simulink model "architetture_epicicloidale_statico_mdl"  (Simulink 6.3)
settings: Solver=ode45  StartTime=0.0  StopTime=3  RelTol=1e-3
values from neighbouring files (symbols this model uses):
  bm = 0.8*N*metri*secondo/rad    (= 0.8)    [architetture_epicicloidale_statico.m]    (also in architetture_HEV_startstop_1.m; architetture_HEV_startstop_2.m = 0.08; architetture_epicicloidale.m; architetture_epicicloidale_cont.m)
  I_m = eye(m-1)    [architetture_epicicloidale_statico.m]    (also in architetture_HEV_startstop_1.m; architetture_HEV_startstop_2.m; architetture_epicicloidale.m; architetture_epicicloidale_cont.m)
  Iw0 = 0*wI0    [architetture_epicicloidale_statico.m]    (also in architetture_HEV_startstop_1.m; architetture_HEV_startstop_2.m; architetture_epicicloidale.m; architetture_epicicloidale_cont.m = wI0)
  Jm = 1.6*kg*metri^2    (= 1.6)    [architetture_epicicloidale_statico.m]    (also in architetture_HEV_startstop_1.m = 0.529459095518; architetture_HEV_startstop_2.m = 0.529459095518; architetture_epicicloidale.m; architetture_epicicloidale_cont.m)
  Jr = Jr([1:m-1],[1:m-1])    [architetture_epicicloidale_statico.m]    (also in architetture_HEV_startstop_1.m; architetture_HEV_startstop_2.m; architetture_epicicloidale.m; architetture_epicicloidale_cont.m)
  Kf = diag(diag(MLb)'./fliplr(tau_m(1:m-1)))    [architetture_epicicloidale_statico.m]    (also in architetture_HEV_startstop_1.m; architetture_HEV_startstop_2.m; architetture_epicicloidale_cont.m; architetture_epicicloidale_HEV.m)
  Kr = Kr([1:m-1])    [architetture_epicicloidale_statico.m]    (also in architetture_HEV_startstop_1.m; architetture_HEV_startstop_2.m; architetture_epicicloidale.m; architetture_epicicloidale_cont.m)
  Li = 0.1*Henry    (= 0.1)    [architetture_epicicloidale_statico.m]    (also in architetture_HEV_startstop_1.m; architetture_HEV_startstop_2.m; architetture_epicicloidale.m; architetture_epicicloidale_cont.m)
  m = 5    [architetture_epicicloidale_statico.m]    (also in architetture_HEV_startstop_1.m; architetture_HEV_startstop_2.m; CVT_New.m = 1; CVT_New_th.m = 1)
  Mi = 0.08*Henry    (= 0.08)    [architetture_epicicloidale_statico.m]    (also in architetture_HEV_startstop_1.m; architetture_HEV_startstop_2.m; architetture_epicicloidale.m; architetture_epicicloidale_cont.m)
  MKr = MKr([1:m-1],[1:m-1])    [architetture_epicicloidale_statico.m]    (also in architetture_HEV_startstop_1.m; architetture_HEV_startstop_2.m; architetture_epicicloidale.m; architetture_epicicloidale_cont.m)
  MLb = MLb([1:m-1],[1:m-1])    [architetture_epicicloidale_statico.m]    (also in architetture_HEV_startstop_1.m; architetture_HEV_startstop_2.m; architetture_epicicloidale.m; architetture_epicicloidale_cont.m)
  MR = MR([1:m-1],[1:m-1])    [architetture_epicicloidale_statico.m]    (also in architetture_HEV_startstop_1.m; architetture_HEV_startstop_2.m; architetture_epicicloidale.m; architetture_epicicloidale_cont.m)
  Nar = 200    [architetture_epicicloidale_statico.m]    (also in architetture_HEV_startstop_1.m; architetture_HEV_startstop_2.m; architetture_epicicloidale.m; architetture_epicicloidale_cont.m)
  Nc = 30    [architetture_epicicloidale_statico.m]    (also in architetture_HEV_startstop_1.m; architetture_HEV_startstop_2.m; architetture_epicicloidale.m; architetture_epicicloidale_cont.m)
  p = 1    [architetture_epicicloidale_statico.m]    (also in architetture_HEV_startstop_1.m; architetture_HEV_startstop_2.m; architetture_epicicloidale.m; architetture_epicicloidale_cont.m)
  Phir = 0.02*Weber    (= 0.02)    [architetture_epicicloidale_statico.m]    (also in architetture_HEV_startstop_1.m; architetture_HEV_startstop_2.m; architetture_epicicloidale.m; architetture_epicicloidale_cont.m)
  r_r = xds*Nr/(2*pi)    (= 0.248281711223)    [architetture_epicicloidale_statico.m]    (also in architetture_HEV_startstop_1.m; architetture_HEV_startstop_2.m; architetture_epicicloidale_HEV.m; architetture_HEV_controllo.m)
  r_s = r_r-2*r_p    (= 0.101859163579)    [architetture_epicicloidale_statico.m]    (also in architetture_HEV_startstop_1.m; architetture_HEV_startstop_2.m; architetture_epicicloidale.m = 0.0732112738223; architetture_epicicloidale_cont.m = 0.0732112738223)
  Ri = 3*Ohm    (= 3)    [architetture_epicicloidale_statico.m]    (also in architetture_HEV_startstop_1.m = 0.1; architetture_HEV_startstop_2.m = 0.1; architetture_epicicloidale.m; architetture_epicicloidale_cont.m)
  Star = Si    [architetture_epicicloidale_statico.m]    (also in architetture_HEV_startstop_1.m; architetture_HEV_startstop_2.m; architetture_epicicloidale.m; architetture_epicicloidale_cont.m)
  Tc = 0.05*ms    (= 5e-05)    [architetture_epicicloidale_statico.m]    (also in architetture_HEV_startstop_1.m; architetture_HEV_startstop_2.m; CVT_New.m; CVT_New_th.m)
  Thm0 = 0    [architetture_epicicloidale_statico.m]    (also in architetture_HEV_startstop_1.m; architetture_HEV_startstop_2.m; architetture_epicicloidale.m; architetture_epicicloidale_cont.m)
  tTb = tTb(:,[1:m-1])    [architetture_epicicloidale_statico.m]    (also in architetture_HEV_startstop_1.m; architetture_HEV_startstop_2.m; architetture_epicicloidale.m; architetture_epicicloidale_cont.m)
  W_ice = 20*rad/secondo    (= 20)    [architetture_epicicloidale_statico.m]
  Wc_0 = -0*0.2*rad/secondo    (= 0)    [architetture_epicicloidale_statico.m]    (also in architetture_epicicloidale.m; architetture_epicicloidale_cont.m; architetture_epicicloidale_HEV.m; architetture_epicicloidale_prova.m)
  Wm0 = 0*Wr_d    (= 0)    [architetture_epicicloidale_statico.m]    (also in architetture_HEV_startstop_1.m; architetture_HEV_startstop_2.m; architetture_epicicloidale.m; architetture_epicicloidale_cont.m = 62.5)
  Wr_0 = WW_0(5),    [CVT_New.m]    (also in CVT_New_th.m; architetture_epicicloidale.m = Sys1.C(3,:)*[Wc_0; Wsc_0]; Confronto_CVT_EMR.m = 0; epicicloidale.m = Sys1.C(3,:)*[Wc_0; Wsc_0])
  Ws_0 = 0*0.1*rad/secondo    (= 0)    [architetture_epicicloidale_statico.m]    (also in epicicloidale_confronto_statico_elastico.m = 0.1; epicicloidale_statico.m = 0.1)
undefined symbols (not defined in the file or in its folder): a_0, a_1, B_Pneumatico, DFKc_max, eps_sk, K_Pneumatico, Lambda_mu, Mass_Matrix, Massa_Corpo_Auto, Mu_lambda, Raggio_Ruota_Ant, Raggio_Ruota_Pos, T_omega, tau_a0
libraries: simulink x11, dspmtrx3 x4, Tire_Soil x2, POG_Sincronous_Motors x1

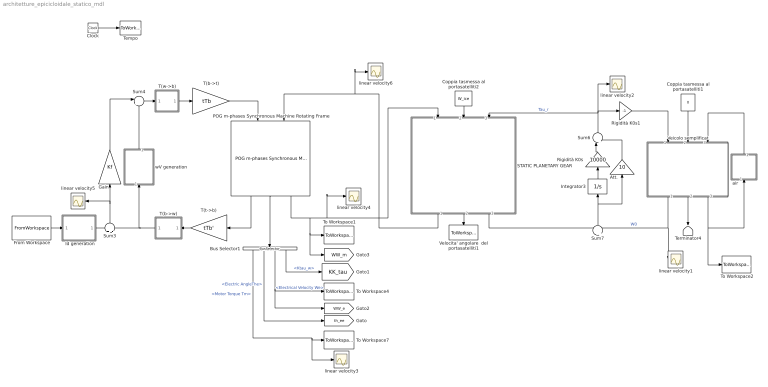
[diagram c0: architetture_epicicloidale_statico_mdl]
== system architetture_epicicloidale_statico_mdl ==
  " Id generation" : Subsystem
  Att. : Gain  Orientation=up  Gain=10
  Bus Selector1 : BusSelector  Orientation=down  OutputSignals=Motor Torque Tm,Electric AngleThe,Electrical Velocity We,Ktau_w
  Clock : Clock
  Coppia tasmessa al portasatelliti1 : Constant  Orientation=down  Value=0
  Coppia tasmessa al portasatelliti2 : Constant  Orientation=down  Value=W_ice
  From Workspace : FromWorkspace  VariableName=[T_in Tau_des]  SampleTime=0
  Gain : Gain  Orientation=up  Gain=Kf  Multiplication=Matrix(K*u) (u vector)
  Integrator3 : Integrator  Orientation=up
  POG m-phases Synchronous Machine Rotating Frame : POG_Sincronous_Motors/POG m-phases Synchronous Machine Rotating Frame  Orientation=down  Motor_Par=[m p]  Phase_Par=[Nc Star]  Electric_Par=[Ri Li Mi]  Mech_Par=[Jm bm]  Plux_Par=[Phir Nar]  Iniz_Cond=[Wm0; Thm0; Iw0]  TipoFlux=User defined  Tipo=Tipo  alfa=al  degree=6  TipoF=Tipo
  Rigidità K0s : Gain  Orientation=up  Gain=10000
  Rigidità K0s1 : Gain  Gain=-1
  STATIC PLANETARY GEAR : Subsystem  Orientation=down  mask(POG Gruppo epicicloidale){Raggi_sun_ring=[r_s, r_r], Tipo_di_Modello=Modello ridotto Ws-Wc, Cond_in_Ws_Wc=[Ws_0,  Wc_0], Cond_in_Wc_Wr=[Wc_0,  Wr_0], Cond_in_Ws_Wr=[Ws_0,  Wr_0], Cond_in=[Ws_0, Wc_0, Wr_0]}
      mask prompts: Raggi_sun_ring "Raggi Sun, Ring: [r_s, r_r]-->[m,m]"; Tipo_di_Modello "Tipo di modello"; Cond_in_Ws_Wc "Condizioni iniziali: [Ws_0,  Wc_0]-->[rad/s]"; Cond_in_Wc_Wr "Condizioni iniziali: [Wc_0,  Wr_0]-->[rad/s]"; Cond_in_Ws_Wr "Condizioni iniziali: [Ws_0,  Wr_0]-->[rad/s]"; Cond_in "Condizioni iniziali: [Ws_0,  Wc_0, Wr_0]-->[rad/s]"
      mask help: Gruppo epicicloidale: [r_s, r_r]= Raggi di: sun e ring; [Ws_0, Wc_0, Wr_0]=Velocita' iniziali di sun, carrieri, ring;
      mask init:
      | r_s=Raggi_sun_ring(1);
      | r_r=Raggi_sun_ring(2);
      | 
      | %
      | %%%%%%%%%%%%%%%%%%%%%%%%%%%%%%%%%%%%%%%%%%%%%%%%%%%%%%%%%%%%%%%%%%%%%%%%%%%
      | %   Modello statico tutti i casi
      | %%%%%%%%%%%%%%%%%%%%%%%%%%%%%%%%%%%%%%%%%%%%%%%%%%%%%%%%%%%%%%%%%%%%%%%%%%%
      | if Tipo_di_Modello=='Modello ridotto Ws-Wc'
      |       %
      |     B= [ -1/r_r*r_s,  (r_s+r_r)/r_r];
      |     %
      |     Ws_0=double(Cond_in_Ws_Wc(1));
      |     Wc_0=double(Cond_in_Ws_Wc(2));
      |     We_0=[Ws_0 Wc_0];
      |     %
      | elseif Tipo_di_Modello=='Modello ridotto Wc-Wr'
      |     B= [ (r_s+r_r)/r_s,  -1/r_s*r_r];
      |    %
      |     Wc_0=double(Cond_in_Wc_Wr(1));
      |     Wr_0=double(Cond_in_Wc_Wr(2));
      |     We_0=[Wc_0 Wr_0];
      |     %
      | elseif Tipo_di_Modello=='Modello ridotto Ws-Wr'
      |  
      |     B=[1/(r_s+r_r)*r_s, 1/(r_s+r_r)*r_r];
      |    %
      |     Ws_0=double(Cond_in_Ws_Wr(1));
      |     Wr_0=double(Cond_in_Ws_Wr(2));
      |     We_0=[Ws_0 Wr_0];
      | end
  Sum3 : Sum  Orientation=up  Inputs=+|-
  Sum4 : Sum  Inputs=|++
  Sum6 : Sum  Orientation=up  Inputs=|++
  Sum7 : Sum  Orientation=up  Inputs=-|+
  T(b->t) : Gain  Gain=tTb  Multiplication=Matrix(K*u) (u vector)
  T(b->w) : Subsystem  Orientation=left  AncestorBlock=|
      | POG_Electric_Bloks/POG m-phases
      | Synchronous Machine
      | Rotating Frame/T(b->w)
  T(t->b) : Gain  Orientation=left  Gain=tTb'  Multiplication=Matrix(K*u) (u vector)
  T(w->b) : Subsystem  AncestorBlock=|
      | POG_Electric_Bloks/POG m-phases
      | Synchronous Machine
      | Rotating Frame/T(w->b)
  Tempo : ToWorkspace  VariableName=t  SampleTime=Tc  SaveFormat=Array
  Terminator4 : Terminator
  To Workspace1 : ToWorkspace  VariableName=Wm  SampleTime=Tc  SaveFormat=Array
  To Workspace2 : ToWorkspace  VariableName=Vvehicle  SampleTime=Tc  SaveFormat=Array
  To Workspace4 : ToWorkspace  VariableName=We  SampleTime=Tc  SaveFormat=Array
  To Workspace7 : ToWorkspace  VariableName=Tm  SampleTime=Tc  SaveFormat=Array
  Veicolo semplificat : Subsystem  Orientation=down
  Velocita' angolare  del portasatelliti1 : ToWorkspace  VariableName=Tau_ice  SampleTime=Tc  SaveFormat=Array
  air : Subsystem  Orientation=up
  linear velocity{1..6} (6 alike) : Scope
  wV generation : Subsystem  Orientation=up
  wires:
  Clock/1 -> Tempo/1
  POG m-phases Synchronous Machine Rotating Frame/3 -> To Workspace1/1, [WW_m], STATIC PLANETARY GEAR/1(W1), linear velocity4/1
  POG m-phases Synchronous Machine Rotating Frame/2 -> Bus Selector1/1
  Bus Selector1/3 -> To Workspace4/1, [WW_e]  "<Electrical Velocity We>"
  T(w->b)/1(It) -> T(b->t)/1
  T(b->t)/1 -> POG m-phases Synchronous Machine Rotating Frame/1
  T(t->b)/1 -> T(b->w)/1(Vt)
  T(b->w)/1(Vw) -> wV generation/1(In1), Sum3/2
  POG m-phases Synchronous Machine Rotating Frame/1 -> T(t->b)/1
  Bus Selector1/2 -> [th_ee]  "<Electric AngleThe>"
  Bus Selector1/1 -> To Workspace7/1, linear velocity3/1  "<Motor Torque Tm>"
  Att./1 -> Sum6/2
  Rigidità K0s/1 -> Sum6/1
  Integrator3/1 -> Rigidità K0s/1
  Sum6/1 -> linear velocity2/1, Rigidità K0s1/1, STATIC PLANETARY GEAR/3(Tau3)  "Tau_r"
  Sum7/1 -> Att./1, Integrator3/1
  Coppia tasmessa al portasatelliti1/1 -> Veicolo semplificat/2(Tau2)
  Rigidità K0s1/1 -> Veicolo semplificat/1(Tau1)
  " Id generation"/1(Out1) -> Sum3/1
  Sum3/1 -> Gain/1, linear velocity5/1
  Sum4/1 -> T(w->b)/1(Iw)
  From Workspace/1 -> " Id generation"/1(In1)
  Gain/1 -> Sum4/1
  wV generation/1(Out1) -> Sum4/2
  Veicolo semplificat/1(W1) -> Sum7/2, linear velocity1/1  "W0"
  Veicolo semplificat/3(V) -> To Workspace2/1, air/1(In1)
  Bus Selector1/4 -> [KK_tau]  "<Ktau_w>"
  air/1(Out1) -> Veicolo semplificat/3(Fres)
  Veicolo semplificat/2(W2) -> Terminator4/1
  Coppia tasmessa al portasatelliti2/1 -> STATIC PLANETARY GEAR/2(W2)
  STATIC PLANETARY GEAR/2(Tau2) -> Velocita' angolare  del portasatelliti1/1
  STATIC PLANETARY GEAR/3(W3) -> Sum7/1
  STATIC PLANETARY GEAR/1(Tau1) -> POG m-phases Synchronous Machine Rotating Frame/2, linear velocity6/1

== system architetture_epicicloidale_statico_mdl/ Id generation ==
  In1 : Inport
  Divide : Product  Inputs=*/  OutScaling=2^-10
  Product : Product
  modulo : Subsystem
  versore : Subsystem
  Out1 : Outport
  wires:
  [KK_tau] -> modulo/1(In1), versore/1(In1)
  modulo/1(Out1) -> Divide/2
  Divide/1 -> Product/1
  versore/1(Out1) -> Product/2
  In1/1 -> Divide/1
  Product/1 -> Out1/1

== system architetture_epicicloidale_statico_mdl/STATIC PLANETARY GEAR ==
  W1 : Inport
  W2 : Inport  Port=2
  Tau3 : Inport  Orientation=left  Port=3
  Demux : Demux  Orientation=left  Outputs=2
  Mux : Mux  Inputs=2
  Rsc : Gain  Gain=B  Multiplication=Matrix(K*u)
  Rsc' : Gain  Orientation=left  Gain=B'  Multiplication=Matrix(K*u)
  Tau1 : Outport  Orientation=left
  Tau2 : Outport  Orientation=left  Port=2
  W3 : Outport  Port=3
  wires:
  Demux/2 -> Tau2/1  "Tau2"
  Demux/1 -> Tau1/1  "Tau1"
  Rsc'/1 -> Demux/1
  Mux/1 -> Rsc/1
  W2/1 -> Mux/2  "W2"
  W1/1 -> Mux/1  "W1"
  Rsc/1 -> W3/1  "W3"
  Tau3/1 -> Rsc'/1  "Tau3"

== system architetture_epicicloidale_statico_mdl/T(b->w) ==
  Vt : Inport
  Product : Product  Multiplication=Matrix(*)
  Vw : Outport
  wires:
  Vt/1 -> Product/2
  Product/1 -> Vw/1
  [T_w_be] -> Product/1

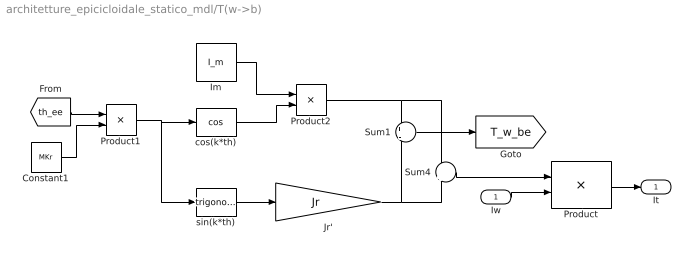
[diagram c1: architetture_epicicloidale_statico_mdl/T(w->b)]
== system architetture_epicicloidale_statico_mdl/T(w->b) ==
  Iw : Inport
  Constant1 : Constant  Value=MKr
  Im : Constant  Value=I_m  VectorParams1D=off
  Jr' : Gain  Gain=Jr  Multiplication=Matrix(K*u)
  Product : Product  Multiplication=Matrix(*)
  Product1 : Product
  Product2 : Product
  Sum1 : Sum  Inputs=+|-
  Sum4 : Sum  Inputs=+|+
  cos(k*th) : Trigonometry  Operator=cos
  sin(k*th) : Trigonometry
  It : Outport
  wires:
  Sum4/1 -> Product/1
  Product/1 -> It/1
  Iw/1 -> Product/2
  Jr'/1 -> Sum4/2, Sum1/2
  Product2/1 -> Sum4/1, Sum1/1
  Im/1 -> Product2/1
  cos(k*th)/1 -> Product2/2
  Product1/1 -> sin(k*th)/1, cos(k*th)/1
  Constant1/1 -> Product1/2
  [th_ee] -> Product1/1
  sin(k*th)/1 -> Jr'/1
  Sum1/1 -> [T_w_be]

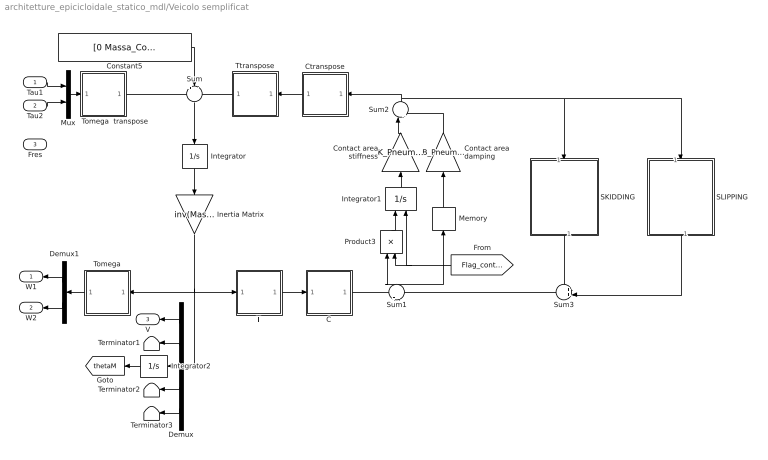
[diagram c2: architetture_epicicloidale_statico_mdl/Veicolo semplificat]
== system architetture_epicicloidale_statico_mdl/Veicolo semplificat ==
  Tau1 : Inport
  Tau2 : Inport  Port=2
  Fres : Inport  Port=3
  C : Subsystem
  Constant5 : Constant  Value=[0 Massa_Corpo_Auto*9.81 0 0 0]
  Contact area damping : Gain  Orientation=up  Gain=B_Pneumatico  Multiplication=Matrix(K*u) (u vector)
  Contact area stiffness : Gain  Orientation=up  Gain=K_Pneumatico  Multiplication=Matrix(K*u) (u vector)
  Ctranspose : Subsystem  Orientation=left
  Demux : Demux  Orientation=left  Outputs=5
  Demux1 : Demux  Orientation=left  Outputs=2
  Inertia Matrix : Gain  Orientation=down  Gain=inv(Mass_Matrix)  Multiplication=Matrix(K*u)
  Integrator : Integrator  Orientation=down  InitialCondition=[0 0 0 0 0]
  Integrator1 : Integrator  Orientation=up  ExternalReset=falling  InitialCondition=[0 0 0 0 0 0]
  Integrator2 : Integrator  Orientation=left
  Memory : Memory  Orientation=up
  Mux : Mux  Inputs=2
  Product3 : Product  Orientation=up  Inputs=**
  SKIDDING : Subsystem  Orientation=down  AncestorBlock=Tire_Soil/Tire-soil contact ENERGETIC/Contatto elastico/SKIDDING
  SLIPPING : Subsystem  Orientation=down  AncestorBlock=Tire_Soil/Tire-soil contact ENERGETIC/Contatto elastico/SLIPPING
  Sum : Sum  Orientation=down  Inputs=+--
  Sum1 : Sum  Orientation=up  Inputs=+-
  Sum2 : Sum  Orientation=up  Inputs=|++
  Sum3 : Sum  Orientation=left  Inputs=++|
  T : Subsystem
  Terminator1 : Terminator
  Terminator2 : Terminator
  Terminator3 : Terminator
  Tomega : Subsystem  Orientation=left
  Tomega  transpose : Subsystem
  Ttranspose : Subsystem  Orientation=left
  W1 : Outport  Orientation=left
  W2 : Outport  Orientation=left  Port=2
  V : Outport  Orientation=left  Port=3
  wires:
  Demux/5 -> Terminator3/1
  Demux/4 -> Terminator2/1
  Demux/2 -> Terminator1/1
  Demux/1 -> V/1
  Tomega/1(Vt) -> Demux1/1
  Tau2/1 -> Mux/2
  Tau1/1 -> Mux/1
  Mux/1 -> Tomega  transpose/1(T)
  Tomega  transpose/1(Tt) -> Sum/1
  Constant5/1 -> Sum/2
  Sum3/1 -> Sum1/2
  SKIDDING/1(Vcsk) -> Sum3/1
  SLIPPING/1(Vcsl) -> Sum3/2
  Memory/1 -> Contact area damping/1
  Integrator1/1 -> Contact area stiffness/1
  Product3/1 -> Integrator1/1
  [Flag_contatto] -> Integrator1/2, Product3/2
  C/1(Xcdot) -> Sum1/1
  Ctranspose/1(F) -> Ttranspose/1(F)
  T/1(Xdot) -> C/1(Xdot)
  Integrator2/1 -> [thetaM]
  Demux/3 -> Integrator2/1
  Contact area stiffness/1 -> Sum2/1
  Contact area damping/1 -> Sum2/2
  Sum1/1 -> Memory/1, Product3/1
  Sum2/1 -> Ctranspose/1(Fc), SLIPPING/1(Fxyz), SKIDDING/1(Fxyz)
  Ttranspose/1(Ft) -> Sum/3
  Inertia Matrix/1 -> T/1(V), Tomega/1(V), Demux/1
  Integrator/1 -> Inertia Matrix/1
  Sum/1 -> Integrator/1
  Demux1/1 -> W1/1
  Demux1/2 -> W2/1

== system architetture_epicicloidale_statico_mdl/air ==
  In1 : Inport  Orientation=up
  air : Fcn  Orientation=up  Expr=10*u^2
  Out1 : Outport  Orientation=up
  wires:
  In1/1 -> air/1
  air/1 -> Out1/1

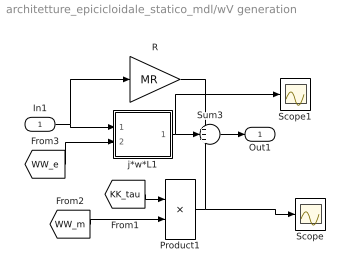
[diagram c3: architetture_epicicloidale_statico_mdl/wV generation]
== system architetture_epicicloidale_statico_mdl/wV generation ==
  In1 : Inport
  Product1 : Product  Multiplication=Matrix(*)
  R : Gain  Gain=MR  Multiplication=Matrix(K*u) (u vector)
  Scope : Scope
  Scope1 : Scope
  Sum3 : Sum  Inputs=+++
  j*w*L1 : Subsystem  AncestorBlock=|
      | POG_Electric_Bloks/POG m-phases
      | Synchronous Machine
      | Rotating Frame/j*w*L
  Out1 : Outport
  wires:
  [KK_tau] -> Product1/1
  [WW_m] -> Product1/2
  R/1 -> Sum3/1
  j*w*L1/1(Out1) -> Sum3/2, Scope1/1
  Product1/1 -> Sum3/3, Scope/1
  In1/1 -> j*w*L1/1(In1), R/1
  Sum3/1 -> Out1/1
  [WW_e] -> j*w*L1/2(In2)

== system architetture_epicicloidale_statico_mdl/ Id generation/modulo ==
  In1 : Inport
  Dot Product : simulink/Math Operations/Dot Product  InputSameDT=on  OutDataType=sfix(16)  OutScaling=2^-10  DoSatur=off
  Math Function : Math  Operator=sqrt
  Out1 : Outport
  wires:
  In1/1 -> Dot Product/1, Dot Product/2
  Dot Product/1 -> Math Function/1
  Math Function/1 -> Out1/1

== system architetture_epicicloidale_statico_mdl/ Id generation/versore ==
  In1 : Inport
  Constant : Constant  Value=0.0001
  Divide : Product  Inputs=*/  OutScaling=2^-10
  Norma  del vettore : Subsystem
  Sum1 : Sum  Inputs=|++
  Out1 : Outport
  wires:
  Divide/1 -> Out1/1  "versore"
  Constant/1 -> Sum1/2
  Sum1/1 -> Divide/2
  Norma  del vettore/1(Out1) -> Sum1/1
  In1/1 -> Norma  del vettore/1(In1), Divide/1

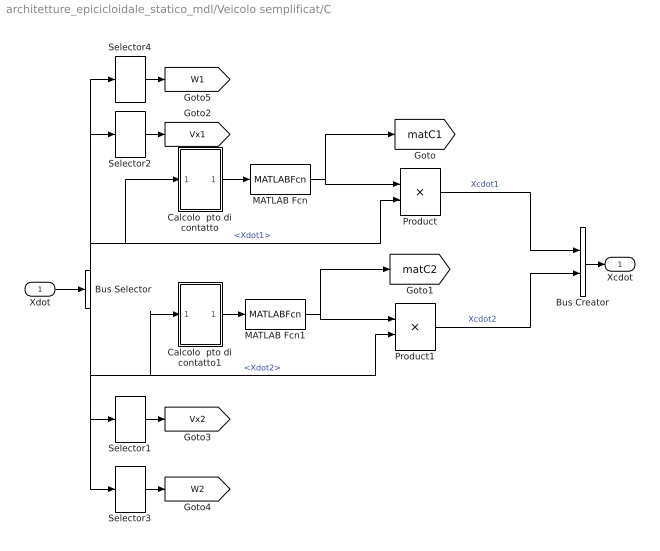
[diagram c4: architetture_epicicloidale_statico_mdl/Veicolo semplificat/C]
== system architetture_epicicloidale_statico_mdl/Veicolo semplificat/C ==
  Xdot : Inport
  Bus Creator : BusCreator  Inputs=2
  Bus Selector : BusSelector  OutputSignals=Xdot1,Xdot2
  Calcolo  pto di contatto : Subsystem
  Calcolo  pto di contatto1 : Subsystem
  MATLAB Fcn : MATLABFcn  MATLABFcn=matrice_c  Output1D=off
  MATLAB Fcn1 : MATLABFcn  MATLABFcn=matrice_c  Output1D=off
  Product : Product  Inputs=**  Multiplication=Matrix(*)
  Product1 : Product  Inputs=**  Multiplication=Matrix(*)
  Selector1 : Selector  InputPortWidth=3
  Selector2 : Selector  InputPortWidth=3
  Selector3 : Selector  Elements=3  InputPortWidth=3
  Selector4 : Selector  Elements=3  InputPortWidth=3
  Xcdot : Outport
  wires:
  Selector3/1 -> [W2]
  Selector4/1 -> [W1]
  Selector1/1 -> [Vx2]
  Selector2/1 -> [Vx1]
  Bus Creator/1 -> Xcdot/1
  Bus Selector/1 -> Selector4/1, Selector2/1, Product/2, Calcolo  pto di contatto/1(In1)  "<Xdot1>"
  Xdot/1 -> Bus Selector/1
  Calcolo  pto di contatto1/1(Out1) -> MATLAB Fcn1/1
  MATLAB Fcn1/1 -> [matC2], Product1/1
  Bus Selector/2 -> Selector3/1, Selector1/1, Calcolo  pto di contatto1/1(In1), Product1/2  "<Xdot2>"
  Product1/1 -> Bus Creator/2  "Xcdot2"
  Calcolo  pto di contatto/1(Out1) -> MATLAB Fcn/1
  MATLAB Fcn/1 -> [matC1], Product/1
  Product/1 -> Bus Creator/1  "Xcdot1"

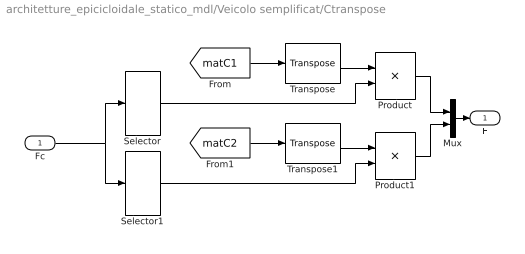
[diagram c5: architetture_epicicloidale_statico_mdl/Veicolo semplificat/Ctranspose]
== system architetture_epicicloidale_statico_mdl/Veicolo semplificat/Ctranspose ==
  Fc : Inport
  Mux : Mux  Inputs=2
  Product : Product  Inputs=**  Multiplication=Matrix(*)
  Product1 : Product  Inputs=**  Multiplication=Matrix(*)
  Selector : Selector  Elements=[1 2 3]  InputPortWidth=6
  Selector1 : Selector  Elements=[4 5 6]  InputPortWidth=6
  Transpose : dspmtrx3/Transpose  Hermitian=off  overflowFlag=on
  Transpose1 : dspmtrx3/Transpose  Hermitian=off  overflowFlag=on
  F : Outport
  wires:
  Selector1/1 -> Product1/2
  Selector/1 -> Product/2
  Fc/1 -> Selector1/1, Selector/1
  Mux/1 -> F/1
  Product1/1 -> Mux/2
  Product/1 -> Mux/1
  [matC2] -> Transpose1/1
  Transpose1/1 -> Product1/1
  [matC1] -> Transpose/1
  Transpose/1 -> Product/1

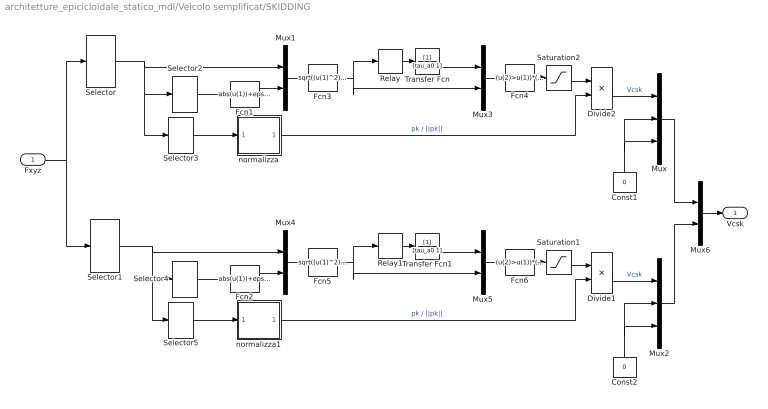
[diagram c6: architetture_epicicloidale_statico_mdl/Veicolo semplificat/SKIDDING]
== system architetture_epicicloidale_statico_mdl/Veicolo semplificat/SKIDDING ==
  Fxyz : Inport
  Const1 : Constant  Orientation=up  Value=0
  Const2 : Constant  Orientation=up  Value=0
  Divide1 : Product  Inputs=**  OutScaling=2^-10
  Divide2 : Product  Inputs=**  OutScaling=2^-10
  Fcn1 : Fcn  Expr=abs(u(1))+eps_sk
  Fcn2 : Fcn  Expr=abs(u(1))+eps_sk
  Fcn3 : Fcn  Expr=sqrt((u(1)^2))/u(4)
  Fcn4 : Fcn  Expr=(u(2)>u(1))*(u(2)-u(1))^2*Kc
  Fcn5 : Fcn  Expr=sqrt((u(1)^2))/u(4)
  Fcn6 : Fcn  Expr=(u(2)>u(1))*(u(2)-u(1))^2*Kc
  Mux : Mux  Inputs=3
  Mux{1,3..6} (5 alike) : Mux  Inputs=2
  Mux2 : Mux  Inputs=3
  Relay : Relay  OnSwitchValue=a_0  OffSwitchValue=a_1  OnOutputValue=a_1  OffOutputValue=a_0
  Relay1 : Relay  OnSwitchValue=a_0  OffSwitchValue=a_1  OnOutputValue=a_1  OffOutputValue=a_0
  Saturation1 : Saturate  UpperLimit=DFKc_max  LowerLimit=0
  Saturation2 : Saturate  UpperLimit=DFKc_max  LowerLimit=0
  Selector : Selector  Elements=[1 2 3]  InputPortWidth=6
  Selector1 : Selector  Elements=[4 5 6]  InputPortWidth=6
  Selector2 : Selector  Elements=[2]  InputPortWidth=3
  Selector3 : Selector  InputPortWidth=3
  Selector4 : Selector  Elements=[2]  InputPortWidth=3
  Selector5 : Selector  InputPortWidth=3
  Transfer Fcn : TransferFcn  Denominator=[tau_a0 1]
  Transfer Fcn1 : TransferFcn  Denominator=[tau_a0 1]
  normalizza : Subsystem
  normalizza1 : Subsystem
  Vcsk : Outport
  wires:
  Mux6/1 -> Vcsk/1
  Mux2/1 -> Mux6/2
  Mux/1 -> Mux6/1
  Const2/1 -> Mux2/3, Mux2/2
  Selector1/1 -> Mux4/1, Selector5/1, Selector4/1
  Divide1/1 -> Mux2/1  "Vcsk"
  Selector4/1 -> Fcn2/1
  Selector5/1 -> normalizza1/1(In1)
  normalizza1/1(Out1) -> Divide1/2  "pk / ||pk||"
  Saturation1/1 -> Divide1/1
  Fcn6/1 -> Saturation1/1
  Fcn5/1 -> Relay1/1, Mux5/2
  Mux4/1 -> Fcn5/1
  Fcn2/1 -> Mux4/2
  Mux5/1 -> Fcn6/1
  Relay1/1 -> Transfer Fcn1/1
  Transfer Fcn1/1 -> Mux5/1
  Const1/1 -> Mux/3, Mux/2
  Selector/1 -> Mux1/1, Selector3/1, Selector2/1
  Divide2/1 -> Mux/1  "Vcsk"
  Fxyz/1 -> Selector1/1, Selector/1
  Selector2/1 -> Fcn1/1
  Selector3/1 -> normalizza/1(In1)
  normalizza/1(Out1) -> Divide2/2  "pk / ||pk||"
  Saturation2/1 -> Divide2/1
  Fcn4/1 -> Saturation2/1
  Fcn3/1 -> Relay/1, Mux3/2
  Mux1/1 -> Fcn3/1
  Fcn1/1 -> Mux1/2
  Mux3/1 -> Fcn4/1
  Relay/1 -> Transfer Fcn/1
  Transfer Fcn/1 -> Mux3/1

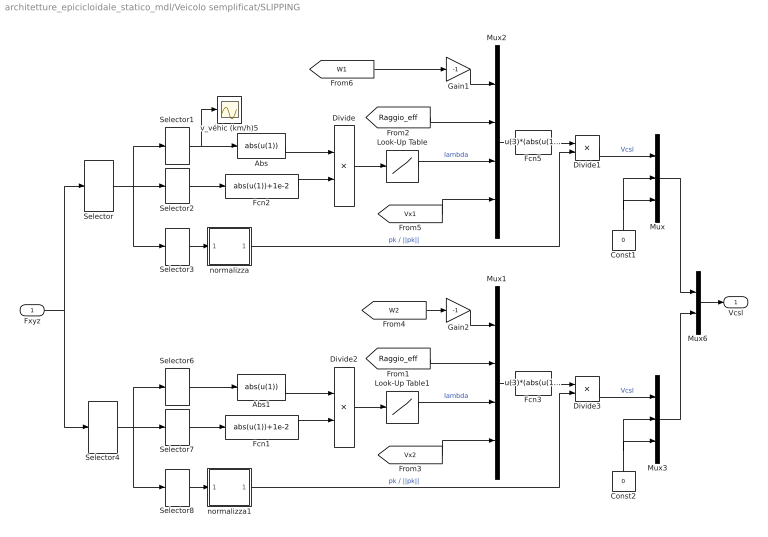
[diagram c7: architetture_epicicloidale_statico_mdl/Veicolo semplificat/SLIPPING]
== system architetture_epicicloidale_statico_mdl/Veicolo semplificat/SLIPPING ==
  Fxyz : Inport
  Abs : Fcn  Expr=abs(u(1))
  Abs1 : Fcn  Expr=abs(u(1))
  Const1 : Constant  Orientation=up  Value=0
  Const2 : Constant  Orientation=up  Value=0
  Divide : Product  Inputs=*/  OutScaling=2^-10
  Divide1 : Product  Inputs=**  OutScaling=2^-10
  Divide2 : Product  Inputs=*/  OutScaling=2^-10
  Divide3 : Product  Inputs=**  OutScaling=2^-10
  Fcn1 : Fcn  Expr=abs(u(1))+1e-2
  Fcn2 : Fcn  Expr=abs(u(1))+1e-2
  Fcn3 : Fcn  Expr=u(3)*(abs(u(1)*u(2))*(abs(u(1)*u(2))<=abs(u(4)))+abs(u(4))*(abs(u(1)*u(2))>abs(u(4))))
  Fcn5 : Fcn  Expr=u(3)*(abs(u(1)*u(2))*(abs(u(1)*u(2))<=abs(u(4)))+abs(u(4))*(abs(u(1)*u(2))>abs(u(4))))
  Gain1 : Gain  Gain=-1
  Gain2 : Gain  Gain=-1
  Look-Up Table : Lookup  InputValues=Mu_lambda  OutputValues=Lambda_mu
  Look-Up Table1 : Lookup  InputValues=Mu_lambda  OutputValues=Lambda_mu
  Mux : Mux  Inputs=3
  Mux1 : Mux
  Mux2 : Mux
  Mux3 : Mux  Inputs=3
  Mux6 : Mux  Inputs=2
  Selector : Selector  Elements=[1 2 3]  InputPortWidth=6
  Selector{1,3,6,8} (4 alike) : Selector  InputPortWidth=3
  Selector2 : Selector  Elements=[2]  InputPortWidth=3
  Selector4 : Selector  Elements=[4 5 6]  InputPortWidth=6
  Selector7 : Selector  Elements=[2]  InputPortWidth=3
  normalizza : Subsystem
  normalizza1 : Subsystem
  v_véhic (km/h)5 : Scope
  Vcsl : Outport
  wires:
  [W2] -> Gain2/1
  [W1] -> Gain1/1
  Mux6/1 -> Vcsl/1
  Mux3/1 -> Mux6/2
  Mux/1 -> Mux6/1
  Const2/1 -> Mux3/3, Mux3/2
  Divide3/1 -> Mux3/1  "Vcsl"
  Const1/1 -> Mux/2, Mux/3
  Divide1/1 -> Mux/1  "Vcsl"
  normalizza1/1(Out1) -> Divide3/2  "pk / ||pk||"
  Selector4/1 -> Selector6/1, Selector8/1, Selector7/1
  Selector7/1 -> Fcn1/1
  Selector8/1 -> normalizza1/1(In1)
  Fcn1/1 -> Divide2/2
  Abs1/1 -> Divide2/1
  Selector6/1 -> Abs1/1
  Look-Up Table1/1 -> Mux1/3  "lambda"
  Divide2/1 -> Look-Up Table1/1
  [Raggio_eff] -> Mux1/2
  Gain2/1 -> Mux1/1
  [Vx2] -> Mux1/4
  Mux1/1 -> Fcn3/1
  Fcn3/1 -> Divide3/1
  Fxyz/1 -> Selector4/1, Selector/1
  normalizza/1(Out1) -> Divide1/2  "pk / ||pk||"
  Selector/1 -> Selector1/1, Selector3/1, Selector2/1
  Selector2/1 -> Fcn2/1
  Selector3/1 -> normalizza/1(In1)
  Fcn2/1 -> Divide/2
  Abs/1 -> Divide/1
  Selector1/1 -> v_véhic (km/h)5/1, Abs/1
  Look-Up Table/1 -> Mux2/3  "lambda"
  Divide/1 -> Look-Up Table/1
  [Raggio_eff] -> Mux2/2
  Gain1/1 -> Mux2/1
  [Vx1] -> Mux2/4
  Mux2/1 -> Fcn5/1
  Fcn5/1 -> Divide1/1

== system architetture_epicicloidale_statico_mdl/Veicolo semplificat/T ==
  V : Inport
  Bus Creator : BusCreator  Inputs=2
  MATLAB Fcn : MATLABFcn  MATLABFcn=matrice_T  Output1D=off
  Product : Product  Inputs=**  Multiplication=Matrix(*)
  Selector : Selector  Elements=[1 2 3]  InputPortWidth=6
  Selector1 : Selector  Elements=[4 5 6]  InputPortWidth=6
  Xdot : Outport
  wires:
  Bus Creator/1 -> Xdot/1
  Selector/1 -> Bus Creator/1  "Xdot1"
  Selector1/1 -> Bus Creator/2  "Xdot2"
  Product/1 -> Selector1/1, Selector/1
  MATLAB Fcn/1 -> [matT], Product/1
  V/1 -> Product/2
  [thetaM] -> MATLAB Fcn/1

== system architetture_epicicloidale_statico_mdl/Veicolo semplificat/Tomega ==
  V : Inport
  Constant5 : Constant  Value=T_omega
  Product : Product  Inputs=**  Multiplication=Matrix(*)
  Vt : Outport
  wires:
  Product/1 -> Vt/1
  V/1 -> Product/2
  Constant5/1 -> Product/1

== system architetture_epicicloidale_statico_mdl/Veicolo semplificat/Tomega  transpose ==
  T : Inport
  Constant5 : Constant  Value=T_omega
  Product : Product  Inputs=**  Multiplication=Matrix(*)
  Transpose : dspmtrx3/Transpose  Hermitian=off  overflowFlag=on
  Tt : Outport
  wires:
  Transpose/1 -> Product/1
  Constant5/1 -> Transpose/1
  T/1 -> Product/2
  Product/1 -> Tt/1

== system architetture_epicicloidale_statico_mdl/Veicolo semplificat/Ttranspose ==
  F : Inport
  Product : Product  Inputs=**  Multiplication=Matrix(*)
  Transpose : dspmtrx3/Transpose  Hermitian=off  overflowFlag=on
  Ft : Outport
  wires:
  Transpose/1 -> Product/1
  [matT] -> Transpose/1
  F/1 -> Product/2
  Product/1 -> Ft/1

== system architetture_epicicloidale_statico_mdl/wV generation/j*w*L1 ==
  In1 : Inport
  In2 : Inport  Port=2
  Gain1 : Gain  Gain=Kr  Multiplication=Matrix(K*u) (u vector)
  Gain2 : Gain  Gain=Jr  Multiplication=Matrix(K*u) (u vector)
  Gain4 : Gain  Gain=MLb  Multiplication=Matrix(K*u) (u vector)
  Product : Product
  Out1 : Outport
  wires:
  In1/1 -> Gain4/1
  In2/1 -> Gain1/1
  Gain1/1 -> Product/1
  Gain4/1 -> Product/2
  Product/1 -> Gain2/1
  Gain2/1 -> Out1/1

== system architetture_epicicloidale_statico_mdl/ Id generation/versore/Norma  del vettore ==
  In1 : Inport
  Dot Product : simulink/Math Operations/Dot Product  InputSameDT=on  OutDataType=sfix(16)  OutScaling=2^-10  DoSatur=off
  Math Function : Math  Operator=sqrt
  Out1 : Outport
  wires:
  Math Function/1 -> Out1/1
  Dot Product/1 -> Math Function/1
  In1/1 -> Dot Product/2, Dot Product/1

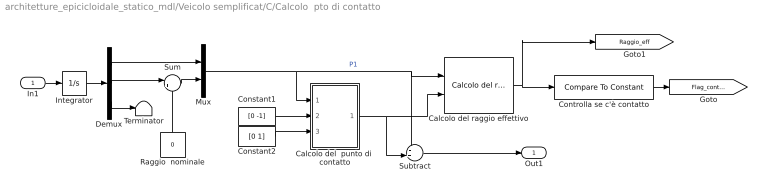
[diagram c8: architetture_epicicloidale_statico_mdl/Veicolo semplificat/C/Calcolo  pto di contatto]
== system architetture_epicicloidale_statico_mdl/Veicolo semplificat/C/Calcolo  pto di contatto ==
  In1 : Inport
  Calcolo del  punto di  contatto : Subsystem  AncestorBlock=|
      | Tire_Soil/Tire-soil contact
      | ENERGETIC/Calcolo versori
      | e punto di contatto C/Subsystem2/Calcolo del 
      | punto di 
      | contatto
  Calcolo del raggio effettivo : Tire_Soil/Tire-soil contact ENERGETIC/Calcolo versori e punto di contatto C/Subsystem2/Calcolo del raggio effettivo
  Constant1 : Constant  Value=[0 -1]
  Constant2 : Constant  Value=[0 1]
  Controlla se c'è contatto : simulink/Logic and Bit Operations/Compare To Constant  relop=<  const=Raggio_Ruota_Ant  LogicOutDataTypeMode=boolean  ZeroCross=off
  Demux : Demux  Outputs=3
  Integrator : Integrator  InitialCondition=[0 Raggio_Ruota_Pos 0]
  Mux : Mux  Inputs=2
  Raggio  nominale : Constant  Orientation=up  Value=0
  Subtract : Sum  Inputs=-+|  OutScaling=2^-10
  Sum : Sum  Inputs=|++
  Terminator : Terminator
  Out1 : Outport
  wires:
  Controlla se c'è contatto/1 -> [Flag_contatto]
  In1/1 -> Integrator/1
  Calcolo del raggio effettivo/1 -> [Raggio_eff], Controlla se c'è contatto/1
  Mux/1 -> Calcolo del  punto di  contatto/1(P1), Calcolo del raggio effettivo/1, Subtract/1  "P1"
  Constant1/1 -> Calcolo del  punto di  contatto/2(r)
  Calcolo del  punto di  contatto/1(Pc) -> Subtract/2, Calcolo del raggio effettivo/2
  Subtract/1 -> Out1/1
  Constant2/1 -> Calcolo del  punto di  contatto/3(n)
  Integrator/1 -> Demux/1
  Sum/1 -> Mux/2
  Demux/1 -> Mux/1
  Raggio  nominale/1 -> Sum/2
  Demux/2 -> Sum/1
  Demux/3 -> Terminator/1

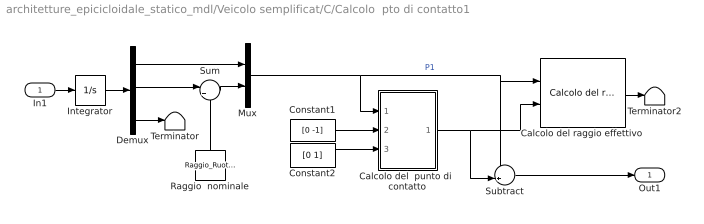
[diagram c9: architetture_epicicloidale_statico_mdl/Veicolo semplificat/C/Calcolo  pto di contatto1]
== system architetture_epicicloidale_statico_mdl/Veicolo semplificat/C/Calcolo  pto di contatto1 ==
  In1 : Inport
  Calcolo del  punto di  contatto : Subsystem  AncestorBlock=|
      | Tire_Soil/Tire-soil contact
      | ENERGETIC/Calcolo versori
      | e punto di contatto C/Subsystem2/Calcolo del 
      | punto di 
      | contatto
  Calcolo del raggio effettivo : Tire_Soil/Tire-soil contact ENERGETIC/Calcolo versori e punto di contatto C/Subsystem2/Calcolo del raggio effettivo
  Constant1 : Constant  Value=[0 -1]
  Constant2 : Constant  Value=[0 1]
  Demux : Demux  Outputs=3
  Integrator : Integrator
  Mux : Mux  Inputs=2
  Raggio  nominale : Constant  Orientation=up  Value=Raggio_Ruota_Pos
  Subtract : Sum  Inputs=-+|  OutScaling=2^-10
  Sum : Sum  Inputs=|++
  Terminator : Terminator
  Terminator2 : Terminator
  Out1 : Outport
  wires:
  In1/1 -> Integrator/1
  Calcolo del raggio effettivo/1 -> Terminator2/1
  Mux/1 -> Calcolo del  punto di  contatto/1(P1), Calcolo del raggio effettivo/1, Subtract/1  "P1"
  Constant1/1 -> Calcolo del  punto di  contatto/2(r)
  Calcolo del  punto di  contatto/1(Pc) -> Calcolo del raggio effettivo/2, Subtract/2
  Subtract/1 -> Out1/1
  Constant2/1 -> Calcolo del  punto di  contatto/3(n)
  Integrator/1 -> Demux/1
  Sum/1 -> Mux/2
  Demux/1 -> Mux/1
  Raggio  nominale/1 -> Sum/2
  Demux/2 -> Sum/1
  Demux/3 -> Terminator/1

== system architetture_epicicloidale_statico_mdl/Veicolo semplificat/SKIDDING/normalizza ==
  In1 : Inport
  Constant : Constant  Value=eps
  Divide : Product  Inputs=*/  OutScaling=2^-10
  Norma  del vettore : Subsystem
  Sum1 : Sum  Inputs=|++
  Out1 : Outport
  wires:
  In1/1 -> Divide/1, Norma  del vettore/1(In1)
  Norma  del vettore/1(Out1) -> Sum1/1
  Sum1/1 -> Divide/2
  Constant/1 -> Sum1/2
  Divide/1 -> Out1/1  "versore"

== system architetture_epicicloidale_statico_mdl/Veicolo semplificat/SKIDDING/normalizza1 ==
  In1 : Inport
  Constant : Constant  Value=eps
  Divide : Product  Inputs=*/  OutScaling=2^-10
  Norma  del vettore : Subsystem
  Sum1 : Sum  Inputs=|++
  Out1 : Outport
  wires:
  In1/1 -> Divide/1, Norma  del vettore/1(In1)
  Norma  del vettore/1(Out1) -> Sum1/1
  Sum1/1 -> Divide/2
  Constant/1 -> Sum1/2
  Divide/1 -> Out1/1  "versore"

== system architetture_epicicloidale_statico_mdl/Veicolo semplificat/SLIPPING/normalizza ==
  In1 : Inport
  Constant : Constant  Value=eps
  Divide : Product  Inputs=*/  OutScaling=2^-10
  Norma  del vettore : Subsystem
  Sum1 : Sum  Inputs=|++
  Out1 : Outport
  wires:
  In1/1 -> Divide/1, Norma  del vettore/1(In1)
  Norma  del vettore/1(Out1) -> Sum1/1
  Sum1/1 -> Divide/2
  Constant/1 -> Sum1/2
  Divide/1 -> Out1/1  "versore"

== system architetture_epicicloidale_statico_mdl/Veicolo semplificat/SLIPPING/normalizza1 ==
  In1 : Inport
  Constant : Constant  Value=eps
  Divide : Product  Inputs=*/  OutScaling=2^-10
  Norma  del vettore : Subsystem
  Sum1 : Sum  Inputs=|++
  Out1 : Outport
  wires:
  In1/1 -> Divide/1, Norma  del vettore/1(In1)
  Norma  del vettore/1(Out1) -> Sum1/1
  Sum1/1 -> Divide/2
  Constant/1 -> Sum1/2
  Divide/1 -> Out1/1  "versore"

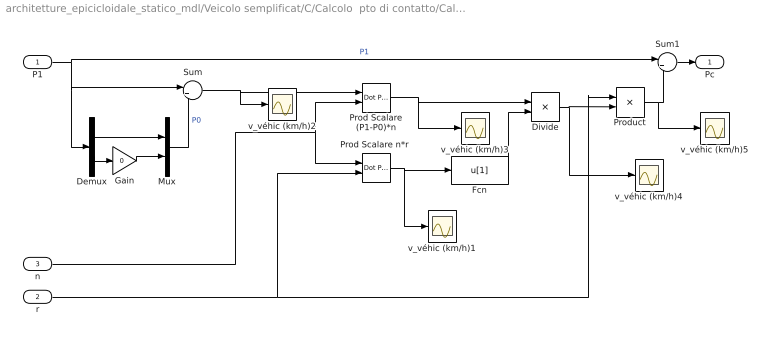
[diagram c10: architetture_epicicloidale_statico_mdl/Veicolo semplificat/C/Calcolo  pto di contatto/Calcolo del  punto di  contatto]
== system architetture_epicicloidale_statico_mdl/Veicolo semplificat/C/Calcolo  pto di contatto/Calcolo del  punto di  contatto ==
  P1 : Inport
  r : Inport  Port=2
  n : Inport  Port=3
  Demux : Demux  Outputs=2
  Divide : Product  Inputs=*/  OutScaling=2^-10
  Fcn : Fcn  Expr=u[1]
  Gain : Gain  Gain=0
  Mux : Mux  Inputs=2
  Prod Scalare (P1-P0)*n : simulink/Math Operations/Dot Product  InputSameDT=on  OutDataType=sfix(16)  OutScaling=2^-10  DoSatur=off
  "Prod Scalare n*r " : simulink/Math Operations/Dot Product  InputSameDT=on  OutDataType=sfix(16)  OutScaling=2^-10  DoSatur=off
  Product : Product
  Sum : Sum  Inputs=|+-
  Sum1 : Sum  Inputs=|+-
  v_véhic (km/h){1..5} (5 alike) : Scope
  Pc : Outport
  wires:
  Gain/1 -> Mux/2
  Mux/1 -> Sum/2  "P0"
  Demux/1 -> Mux/1
  Demux/2 -> Gain/1
  P1/1 -> Demux/1, Sum/1, Sum1/1  "P1"
  r/1 -> "Prod Scalare n*r "/2, Product/1
  Prod Scalare (P1-P0)*n/1 -> v_véhic (km/h)3/1, Divide/1
  "Prod Scalare n*r "/1 -> v_véhic (km/h)1/1, Fcn/1
  Divide/1 -> v_véhic (km/h)4/1, Product/2
  Product/1 -> v_véhic (km/h)5/1, Sum1/2
  Sum1/1 -> Pc/1
  Sum/1 -> v_véhic (km/h)2/1, Prod Scalare (P1-P0)*n/1
  Fcn/1 -> Divide/2
  n/1 -> "Prod Scalare n*r "/1, Prod Scalare (P1-P0)*n/2

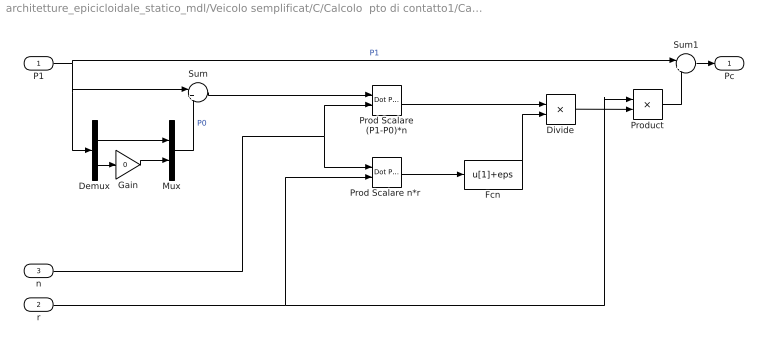
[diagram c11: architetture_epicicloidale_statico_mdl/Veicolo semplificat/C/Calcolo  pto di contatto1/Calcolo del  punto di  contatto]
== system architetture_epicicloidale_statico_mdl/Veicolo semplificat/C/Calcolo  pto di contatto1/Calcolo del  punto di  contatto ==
  P1 : Inport
  r : Inport  Port=2
  n : Inport  Port=3
  Demux : Demux  Outputs=2
  Divide : Product  Inputs=*/  OutScaling=2^-10
  Fcn : Fcn  Expr=u[1]+eps
  Gain : Gain  Gain=0
  Mux : Mux  Inputs=2
  Prod Scalare (P1-P0)*n : simulink/Math Operations/Dot Product  InputSameDT=on  OutDataType=sfix(16)  OutScaling=2^-10  DoSatur=off
  "Prod Scalare n*r " : simulink/Math Operations/Dot Product  InputSameDT=on  OutDataType=sfix(16)  OutScaling=2^-10  DoSatur=off
  Product : Product
  Sum : Sum  Inputs=|+-
  Sum1 : Sum  Inputs=|+-
  Pc : Outport
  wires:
  Gain/1 -> Mux/2
  Mux/1 -> Sum/2  "P0"
  Demux/1 -> Mux/1
  Demux/2 -> Gain/1
  P1/1 -> Demux/1, Sum/1, Sum1/1  "P1"
  r/1 -> "Prod Scalare n*r "/2, Product/1
  Prod Scalare (P1-P0)*n/1 -> Divide/1
  "Prod Scalare n*r "/1 -> Fcn/1
  Divide/1 -> Product/2
  Product/1 -> Sum1/2
  Sum1/1 -> Pc/1
  Sum/1 -> Prod Scalare (P1-P0)*n/1
  Fcn/1 -> Divide/2
  n/1 -> "Prod Scalare n*r "/1, Prod Scalare (P1-P0)*n/2

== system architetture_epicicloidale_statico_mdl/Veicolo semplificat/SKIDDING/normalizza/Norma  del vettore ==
  In1 : Inport
  Dot Product : simulink/Math Operations/Dot Product  InputSameDT=on  OutDataType=sfix(16)  OutScaling=2^-10  DoSatur=off
  Math Function : Math  Operator=sqrt
  Out1 : Outport
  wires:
  In1/1 -> Dot Product/1, Dot Product/2
  Dot Product/1 -> Math Function/1
  Math Function/1 -> Out1/1

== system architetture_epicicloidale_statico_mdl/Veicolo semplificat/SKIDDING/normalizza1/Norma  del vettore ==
  In1 : Inport
  Dot Product : simulink/Math Operations/Dot Product  InputSameDT=on  OutDataType=sfix(16)  OutScaling=2^-10  DoSatur=off
  Math Function : Math  Operator=sqrt
  Out1 : Outport
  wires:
  In1/1 -> Dot Product/1, Dot Product/2
  Dot Product/1 -> Math Function/1
  Math Function/1 -> Out1/1

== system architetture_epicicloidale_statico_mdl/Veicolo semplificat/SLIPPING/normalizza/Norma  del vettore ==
  In1 : Inport
  Dot Product : simulink/Math Operations/Dot Product  InputSameDT=on  OutDataType=sfix(16)  OutScaling=2^-10  DoSatur=off
  Math Function : Math  Operator=sqrt
  Out1 : Outport
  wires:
  In1/1 -> Dot Product/1, Dot Product/2
  Dot Product/1 -> Math Function/1
  Math Function/1 -> Out1/1

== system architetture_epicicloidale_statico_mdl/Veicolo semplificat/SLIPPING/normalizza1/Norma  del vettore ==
  In1 : Inport
  Dot Product : simulink/Math Operations/Dot Product  InputSameDT=on  OutDataType=sfix(16)  OutScaling=2^-10  DoSatur=off
  Math Function : Math  Operator=sqrt
  Out1 : Outport
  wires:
  In1/1 -> Dot Product/1, Dot Product/2
  Dot Product/1 -> Math Function/1
  Math Function/1 -> Out1/1
